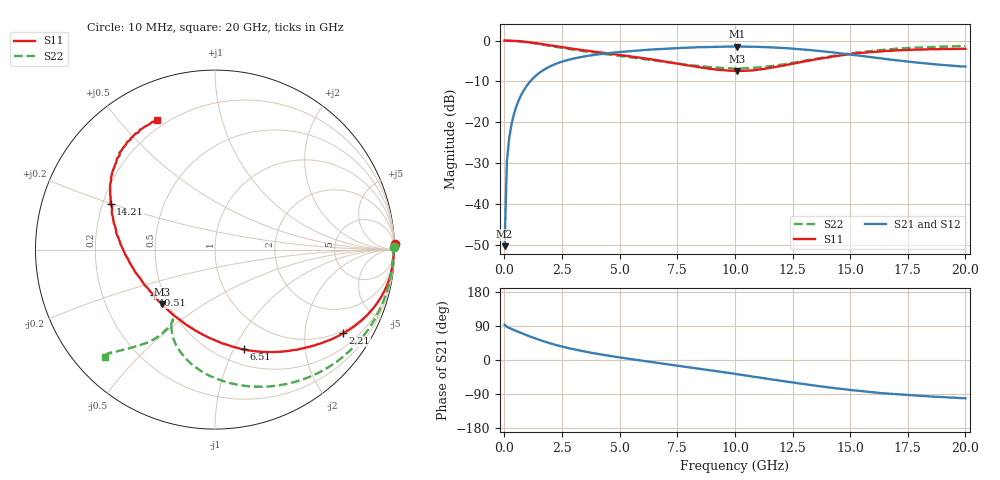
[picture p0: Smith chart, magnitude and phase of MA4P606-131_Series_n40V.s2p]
! AWR Design Environment (9226) Thu Aug 19 15:24:37 2021
! Document = 'n40V'
! nPorts: 2, nXvals: 201
# GHz S DB R 50
!Freq DBS11 AngS11 DBS21 AngS21 DBS12 AngS12 DBS22 AngS22
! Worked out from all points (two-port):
!   201 points, 10 MHz to 20 GHz, reference 50 ohm
!   highest |S21| = -1.48 dB at 10.11 GHz (marker M1); lowest = -50.4 dB at 10 MHz (marker M2)
!   |S21| within 3 dB of the highest: 2.955 GHz to 16.49 GHz (13.53 GHz wide, 139 % of centre)
!   lowest |S11| = -7.5 dB at 10.11 GHz (marker M3), VSWR 2.47, Z = 23.2 - j17.2 ohm
!   |S11| at or under -10 dB: nowhere
!   |S22| runs from -6.9 to 0.0 dB; largest |S21 - S12| = 0.024
!   S11 on the Smith chart (normalised r, x): 10 MHz: -4, +64; 2.21 GHz: 0.91, -3.12; 6.51 GHz: 0.66, -1.10; 10.51 GHz: 0.44, -0.27; 14.21 GHz: 0.23, +0.20; 20 GHz: 0.17, +0.63
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0.01  0.02 1.8  -50.38 93.0  -50.06 80.9  -0.02 1.0
0.11  -0.04 -1.7  -29.48 87.3  -29.47 86.9  -0.07 -3.8
0.21  -0.06 -3.7  -23.87 84.4  -23.89 84.3  -0.08 -7.2
0.41  -0.09 -7.2  -18.14 79.2  -18.14 79.2  -0.13 -14.0
0.71  -0.20 -12.3  -13.56 71.7  -13.56 71.8  -0.26 -23.8
1.11  -0.45 -18.7  -10.09 62.0  -10.09 62.3  -0.53 -36.3
1.61  -0.85 -25.8  -7.55 51.2  -7.54 51.5  -0.96 -50.2
2.21  -1.37 -33.1  -5.77 40.1  -5.76 40.6  -1.53 -64.3
3.41  -2.36 -44.9  -3.96 23.1  -3.94 23.8  -2.59 -84.9
4.81  -3.39 -57.2  -2.92 8.5  -2.90 9.3  -3.64 -100.5
6.51  -4.75 -73.8  -2.16 -6.3  -2.11 -5.4  -4.89 -112.7
6.71  -4.91 -76.0  -2.09 -8.0  -2.04 -7.1  -5.04 -113.8
8.41  -6.50 -100.1  -1.65 -22.4  -1.60 -21.4  -6.24 -119.9
10.01  -7.45 -131.9  -1.48 -36.7  -1.43 -35.3  -6.86 -121.1
10.11  -7.45 -134.1  -1.48 -37.5  -1.43 -36.2  -6.85 -121.0
10.51  -7.41 -143.3  -1.49 -41.2  -1.44 -39.8  -6.81 -120.9
11.91  -6.32 -172.0  -1.78 -54.1  -1.69 -52.6  -6.00 -120.7
13.41  -4.71 165.6  -2.42 -66.9  -2.31 -65.6  -4.57 -123.6
14.21  -3.96 156.5  -2.89 -73.3  -2.76 -72.0  -3.83 -126.2
16.71  -2.55 136.1  -4.64 -89.0  -4.59 -87.9  -2.15 -133.7
19.01  -2.06 122.1  -5.96 -97.8  -6.08 -97.3  -1.50 -135.9
20  -2.05 114.3  -6.37 -101.2  -6.56 -100.1  -1.33 -135.5
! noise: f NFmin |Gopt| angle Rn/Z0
0.01  0  1  0  2e-20
2.21  0  1  0  2e-20
4.41  0  1  0  2e-20
6.61  0  1  0  2e-20
8.81  0  1  0  2e-20
11.11  0  1  0  2e-20
13.31  0  1  0  2e-20
15.51  0  1  0  2e-20
17.71  0  1  0  2e-20
20  0  1  0  2e-20
